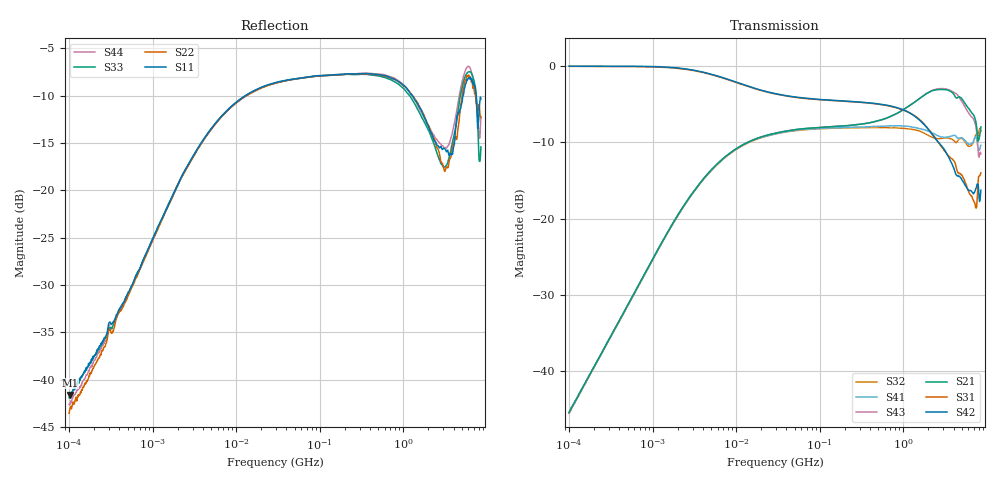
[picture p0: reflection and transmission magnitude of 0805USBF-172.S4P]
# Hz S dB R 50
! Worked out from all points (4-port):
!   801 points, 100 kHz to 8.5 GHz, reference 50 ohm
!   strongest paths, dB at 100 kHz, 1.721 MHz, 29.51 MHz, 502.3 MHz, 8.5 GHz:
!     S42: 0.0, -0.2, -3.6, -5.0, -16.3
!     S31: 0.0, -0.2, -3.7, -5.0, -14.0
!     S21: -45.4, -20.7, -8.8, -7.2, -8.0
!     S43: -45.5, -20.7, -8.8, -7.2, -11.5
!     S41: -45.4, -20.7, -8.9, -7.9, -10.4
!     S32: -45.5, -20.8, -8.9, -8.1, -8.6
!   lowest |S11| = -41.6 dB at 101.7 kHz (marker M1), VSWR 1.02, Z = 50.3 + j0.792 ohm
!   |S11| at or under -10 dB: start of sweep to 12.8 MHz; 1.289 GHz to 5.204 GHz (3.914 GHz wide, 121 % of centre); 7.466 GHz to end of sweep
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100000  -41.52 72.0  -45.38 87.9  -0.05 -0.4  -45.46 -91.7
        -45.37 88.4  -43.56 63.3  -45.57 -91.4  -0.03 -0.3
        -0.05 -0.4  -45.49 -91.9  -41.91 54.2  -45.39 88.4
        -45.44 -91.5  -0.03 -0.3  -45.49 88.4  -42.62 70.4
101665  -41.63 71.8  -45.20 88.5  -0.05 -0.4  -45.31 -91.7
        -45.18 87.9  -43.18 62.9  -45.34 -91.5  -0.02 -0.3
        -0.05 -0.4  -45.33 -92.4  -41.74 53.8  -45.21 88.1
        -45.26 -91.8  -0.03 -0.3  -45.27 88.6  -42.66 71.0
1.046287e7  -10.55 32.9  -10.70 33.3  -2.23 -14.4  -10.76 -147.5
            -10.71 33.4  -10.60 33.0  -10.81 -147.4  -2.19 -14.4
            -2.24 -14.4  -10.80 -147.4  -10.57 32.7  -10.72 33.3
            -10.75 -147.5  -2.19 -14.4  -10.70 33.4  -10.61 33.3
1.823651e9  -12.41 47.6  -3.77 85.2  -7.76 15.6  -8.39 178.2
            -3.76 85.1  -12.32 58.8  -8.86 -178.4  -7.80 13.7
            -7.76 15.5  -8.86 -178.5  -12.92 57.2  -3.73 84.6
            -8.38 178.2  -7.79 13.8  -3.73 84.6  -12.51 47.5
2.843154e9  -15.38 -97.2  -3.07 -87.8  -10.50 -166.6  -9.31 -11.0
            -3.07 -87.9  -17.00 -93.1  -9.47 -3.5  -10.42 -170.1
            -10.52 -166.7  -9.48 -3.6  -17.21 -92.8  -2.95 -89.3
            -9.31 -10.9  -10.40 -170.1  -2.95 -89.3  -15.17 -106.9
3.88629e9  -16.20 125.7  -3.50 96.4  -12.18 2.8  -9.13 161.9
           -3.50 96.2  -15.34 111.6  -9.64 167.0  -13.03 -4.9
           -12.21 2.6  -9.63 167.0  -14.92 132.0  -3.35 94.5
           -9.13 161.9  -13.02 -4.9  -3.35 94.6  -13.83 117.6
8.5e9  -10.36 83.9  -7.96 78.2  -13.93 -141.1  -10.52 70.4
       -7.97 78.4  -12.30 112.1  -8.62 76.3  -16.21 -137.8
       -14.01 -141.8  -8.57 76.7  -15.40 106.0  -11.52 70.3
       -10.39 70.4  -16.28 -138.0  -11.51 70.3  -12.22 78.4
